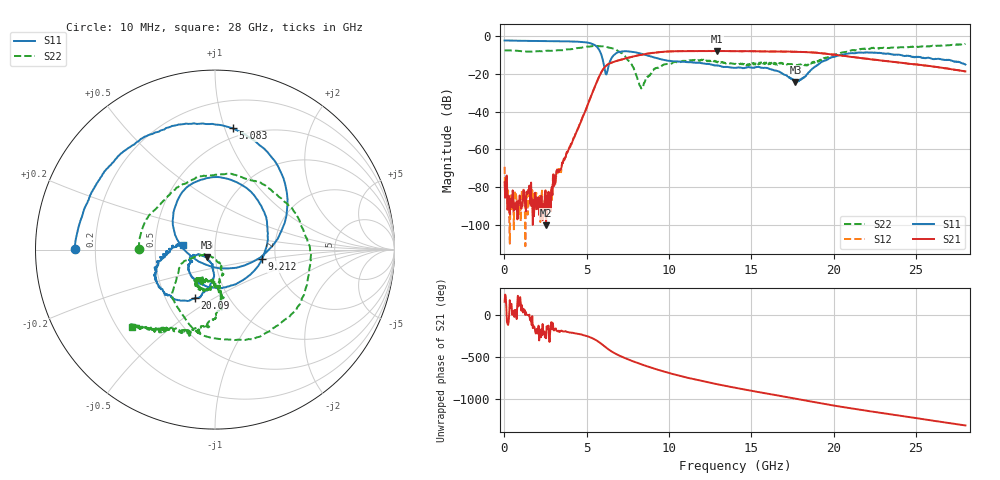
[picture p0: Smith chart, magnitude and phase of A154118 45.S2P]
!  2-Port S-parameters saved by WinCal
! VAR MeasName=S-Parameters (CALIBRATED_DATA) read from VNA (N5230A)
! VAR MeasDate=2015-9-10 14:37:57
! VAR NAME=A154118 45
! VAR FILENAME=A154118 45.S2P
! VAR DATE=2015-9-10 14:37:57
! VAR PHYS_PORTS=1,2
# Hz S DB R 50
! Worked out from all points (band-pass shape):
!   801 points, 10 MHz to 28 GHz, reference 50 ohm
!   highest |S21| = -7.74 dB at 12.89 GHz (marker M1); lowest = -100.3 dB at 2.529 GHz (marker M2)
!   |S21| within 3 dB of the highest: 7.788 GHz to 20.95 GHz (13.16 GHz wide, 91.6 % of centre)
!   lowest |S11| = -24.2 dB at 17.68 GHz (marker M3), VSWR 1.13, Z = 45.5 - j3.89 ohm
!   |S11| at or under -10 dB: 5.895 GHz to 6.639 GHz (744.5 MHz wide, 11.9 % of centre); 8.632 GHz to 20.33 GHz (11.69 GHz wide, 80.8 % of centre); 24.14 GHz to end of sweep
!   |S22| runs from -27.6 to -4.0 dB; largest |S21 - S12| = 0.0072
!   S11 on the Smith chart (normalised r, x): 10 MHz: 0.12, +0.00; 5.083 GHz: 0.42, +1.07; 9.212 GHz: 1.70, -0.19; 20.09 GHz: 0.70, -0.41; 28 GHz: 0.70, +0.04
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1e7  -2.15 179.7  -77.50 149.9  -69.23 154.5  -7.50 179.8
2.549125e8  -2.18 176.2  -84.52 -86.3  -87.50 -66.1  -7.45 172.1
2.5291e9  -2.46 145.9  -100.32 80.6  -97.24 -67.4  -7.63 104.8
2.94895e9  -2.53 139.2  -76.56 -119.5  -73.38 -134.6  -7.59 89.7
4.698325e9  -3.01 98.2  -44.04 124.1  -43.94 122.9  -5.94 12.5
5.083188e9  -3.31 81.6  -35.70 101.6  -35.64 101.5  -5.34 -7.5
5.712962e9  -6.62 30.4  -22.07 39.5  -22.05 39.2  -5.15 -44.1
6.237775e9  -18.95 -143.9  -15.14 -39.1  -15.13 -39.3  -5.71 -75.4
6.86755e9  -8.53 117.2  -12.86 -113.1  -12.86 -113.1  -7.56 -113.2
7.70725e9  -8.14 70.1  -10.91 176.6  -10.91 176.5  -14.72 -159.6
8.302038e9  -9.20 39.2  -9.75 133.9  -9.74 133.7  -27.62 -132.1
9.211712e9  -11.45 -11.1  -8.54 76.0  -8.54 75.7  -16.76 -70.8
9.351662e9  -11.76 -20.0  -8.45 67.7  -8.40 67.5  -16.69 -74.6
1.082114e10  -13.39 -97.0  -7.83 -10.4  -7.79 -11.0  -13.08 -97.3
1.28854e10  -15.43 -149.9  -7.74 -99.3  -7.72 -100.0  -13.27 -118.6
1.4005e10  -16.68 -153.8  -7.85 -142.0  -7.83 -142.4  -14.60 -121.1
1.56844e10  -16.63 -160.0  -7.97 158.1  -7.99 157.6  -13.68 -110.7
1.767869e10  -24.18 -136.5  -8.16 88.9  -8.14 88.7  -14.96 -105.2
1.869332e10  -17.19 -92.2  -8.51 53.4  -8.54 53.0  -13.67 -87.2
2.009282e10  -10.67 -112.8  -9.76 5.2  -9.77 4.5  -9.58 -84.6
2.334666e10  -9.25 -162.7  -13.18 -92.2  -13.22 -93.0  -6.19 -115.2
2.8e10  -14.94 172.1  -18.56 133.6  -18.61 133.0  -3.99 -136.9
